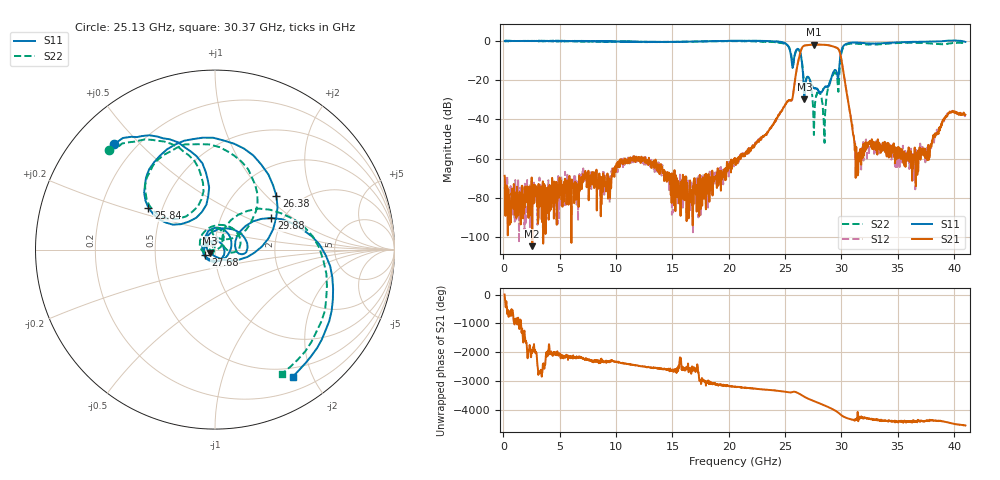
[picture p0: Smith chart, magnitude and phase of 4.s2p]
!The following data was pulled from an Agilent PNA
!This sNp file was generated from the data in the RF Test software
!NOTE:  Smoothing/Math/Corrections applied on any given trace ARE included in the data saved here
# MHz S dB R 50
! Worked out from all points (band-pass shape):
!   1601 points, 100 MHz to 41 GHz, reference 50 ohm
!   highest |S21| = -1.80 dB at 27.58 GHz (marker M1); lowest = -104.6 dB at 2.554 GHz (marker M2)
!   |S21| within 3 dB of the highest: 26.4 GHz to 29.79 GHz (3.388 GHz wide, 12.1 % of centre)
!   lowest |S11| = -29.8 dB at 26.71 GHz (marker M3), VSWR 1.07, Z = 47.4 - j1.77 ohm
!   |S11| at or under -10 dB: 25.58 GHz to 25.77 GHz (189.1 MHz wide, 0.737 % of centre); 26.47 GHz to 29.86 GHz (3.387 GHz wide, 12 % of centre)
!   |S22| runs from -51.9 to 0.2 dB; largest |S21 - S12| = 0.0069
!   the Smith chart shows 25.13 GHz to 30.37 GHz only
!   S11 on the Smith chart (normalised r, x): 25.13 GHz: 0.12, +0.42; 25.84 GHz: 0.42, +0.24; 26.38 GHz: 1.51, +1.15; 27.68 GHz: 0.90, -0.06; 29.88 GHz: 1.74, +0.70; 30.37 GHz: 0.38, -1.72
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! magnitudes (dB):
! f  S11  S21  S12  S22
! 100 MHz  0.0  -68.7  -74.4  0.0
! 2.554 GHz  0.1  -104.6  -82.7  -0.1
! 6.925 GHz  -0.1  -69.3  -68.4  -0.2
! 13.75 GHz  -0.5  -65.2  -61.8  -0.5
! 16.59 GHz  -0.3  -79.6  -72.4  -0.3
! 20.55 GHz  0.1  -59.6  -61.6  -0.1
! 25.13 GHz  -1.8  -31.5  -31.3  -1.8
! 25.84 GHz  -7.2  -21.4  -21.3  -7.8
! 26.38 GHz  -6.8  -5.3  -5.3  -6.9
! 26.71 GHz  -29.8  -2.4  -2.3  -23.4
! 27.38 GHz  -22.6  -1.9  -1.8  -26.3
! 27.58 GHz  -23.9  -1.8  -1.8  -41.4
! 27.68 GHz  -24.0  -1.8  -1.8  -30.6
! 28.01 GHz  -26.1  -1.9  -1.9  -25.7
! 28.5 GHz  -23.8  -1.9  -2.0  -51.9
! 29.88 GHz  -8.9  -6.4  -6.4  -11.0
! 30.37 GHz  -1.6  -22.9  -23.0  -2.1
! 31.41 GHz  -0.9  -58.7  -61.7  -1.5
! 34.2 GHz  -1.0  -59.4  -53.4  -1.3
! 36.6 GHz  -0.4  -74.0  -61.1  -0.9
! 39.47 GHz  0.2  -37.4  -37.2  -1.4
! 41 GHz  -0.5  -37.6  -37.9  -1.1
